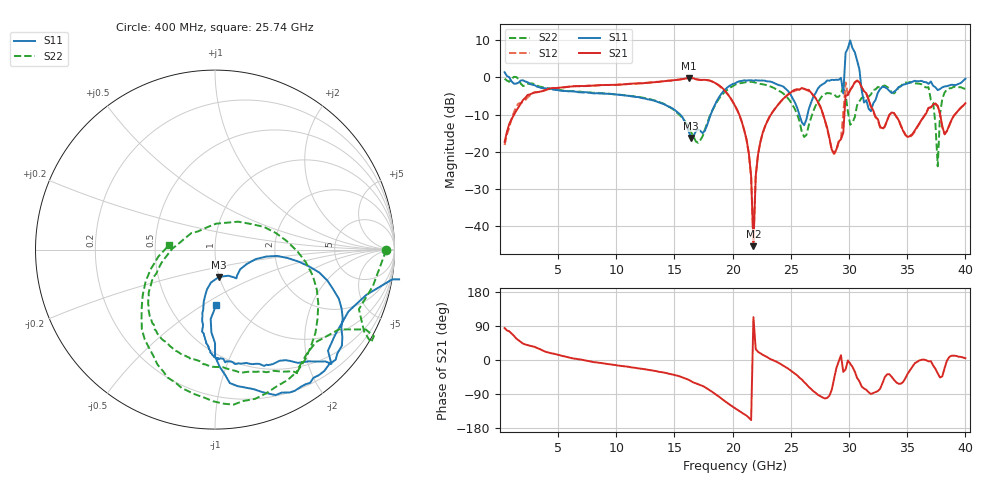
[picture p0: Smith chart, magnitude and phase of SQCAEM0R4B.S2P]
! Network Analyzer HP8722ES.07.66: Jul 25, 2000 Serial No. US39175408
! 26 Oct 2004  08:48:58
! Frequency  S11  S21  S12  S22
# HZ  S  DB R  50
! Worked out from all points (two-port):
!   201 points, 400 MHz to 40 GHz, reference 50 ohm
!   highest |S21| = -0.23 dB at 16.24 GHz (marker M1); lowest = -45.3 dB at 21.78 GHz (marker M2)
!   |S21| within 3 dB of the highest: 4.085 GHz to 19.22 GHz (15.13 GHz wide, 130 % of centre); 30.14 GHz to 31.19 GHz (1.055 GHz wide, 3.44 % of centre)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
!   lowest |S11| = -16.3 dB at 16.44 GHz (marker M3), VSWR 1.36, Z = 49.8 - j15.5 ohm
!   |S11| at or under -10 dB: 15.48 GHz to 18.12 GHz (2.633 GHz wide, 15.7 % of centre); 25.73 GHz to 26.43 GHz (707.6 MHz wide, 2.71 % of centre)
!   |S22| runs from -23.9 to 0.1 dB; largest |S21 - S12| = 0.3
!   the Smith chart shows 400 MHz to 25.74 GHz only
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4e8  1.34 -6.0  -17.32 84.3  -18.17 88.2  -0.41 -0.1
7.132e9  -4.08 -84.1  -2.36 0.1  -2.41 -0.9  -4.04 -97.5
1.3666e10  -6.72 -99.1  -1.27 -31.3  -1.21 -31.3  -6.64 -143.0
1.624e10  -14.67 -97.0  -0.23 -52.8  -0.22 -53.4  -13.57 172.0
1.6438e10  -16.26 -81.8  -0.25 -56.1  -0.21 -56.3  -14.81 161.0
2.02e10  -1.65 -31.7  -7.67 -127.3  -7.63 -128.4  -2.02 -50.7
2.1388e10  -0.82 -47.9  -20.35 -152.3  -20.49 -153.9  -1.33 -79.4
2.1784e10  -0.91 -52.5  -45.28 113.0  -44.08 102.8  -1.31 -86.9
2.2774e10  -0.94 -62.5  -13.22 10.6  -13.32 10.0  -2.01 -103.5
2.6932e10  -5.25 -21.7  -4.89 -82.2  -4.90 -83.3  -9.07 18.8
2.9308e10  -0.17 -20.7  -16.64 12.8  -16.52 12.3  -4.45 -44.6
2.9506e10  -4.36 29.4  -14.89 -31.5  -9.75 -16.2  -2.28 83.7
2.9704e10  6.52 -56.5  -4.97 -25.0  -1.41 -17.0  -4.65 -148.8
3.01e10  9.85 -66.8  -3.40 -9.4  -3.45 -10.1  -12.75 -79.7
3.0496e10  6.70 -84.4  -1.36 -30.6  -1.36 -31.1  -10.69 -59.1
3.0694e10  4.46 73.5  -0.95 -47.4  -0.87 -48.1  -7.47 127.6
3.1288e10  -6.78 69.7  -3.74 -75.2  -3.90 -76.8  -5.37 120.2
3.1486e10  -6.15 -88.6  -4.29 -78.8  -4.48 -80.2  -4.95 -62.4
3.3466e10  -3.66 -38.3  -10.08 -37.4  -10.10 -38.2  -3.10 -90.1
3.6832e10  -1.78 -67.6  -8.20 -3.5  -8.23 -4.6  -2.68 -109.6
3.7624e10  -3.43 -67.2  -7.65 -35.3  -7.85 -35.9  -23.87 -35.2
4e10  -0.41 -57.0  -6.96 4.8  -7.16 5.4  -3.14 -78.1
